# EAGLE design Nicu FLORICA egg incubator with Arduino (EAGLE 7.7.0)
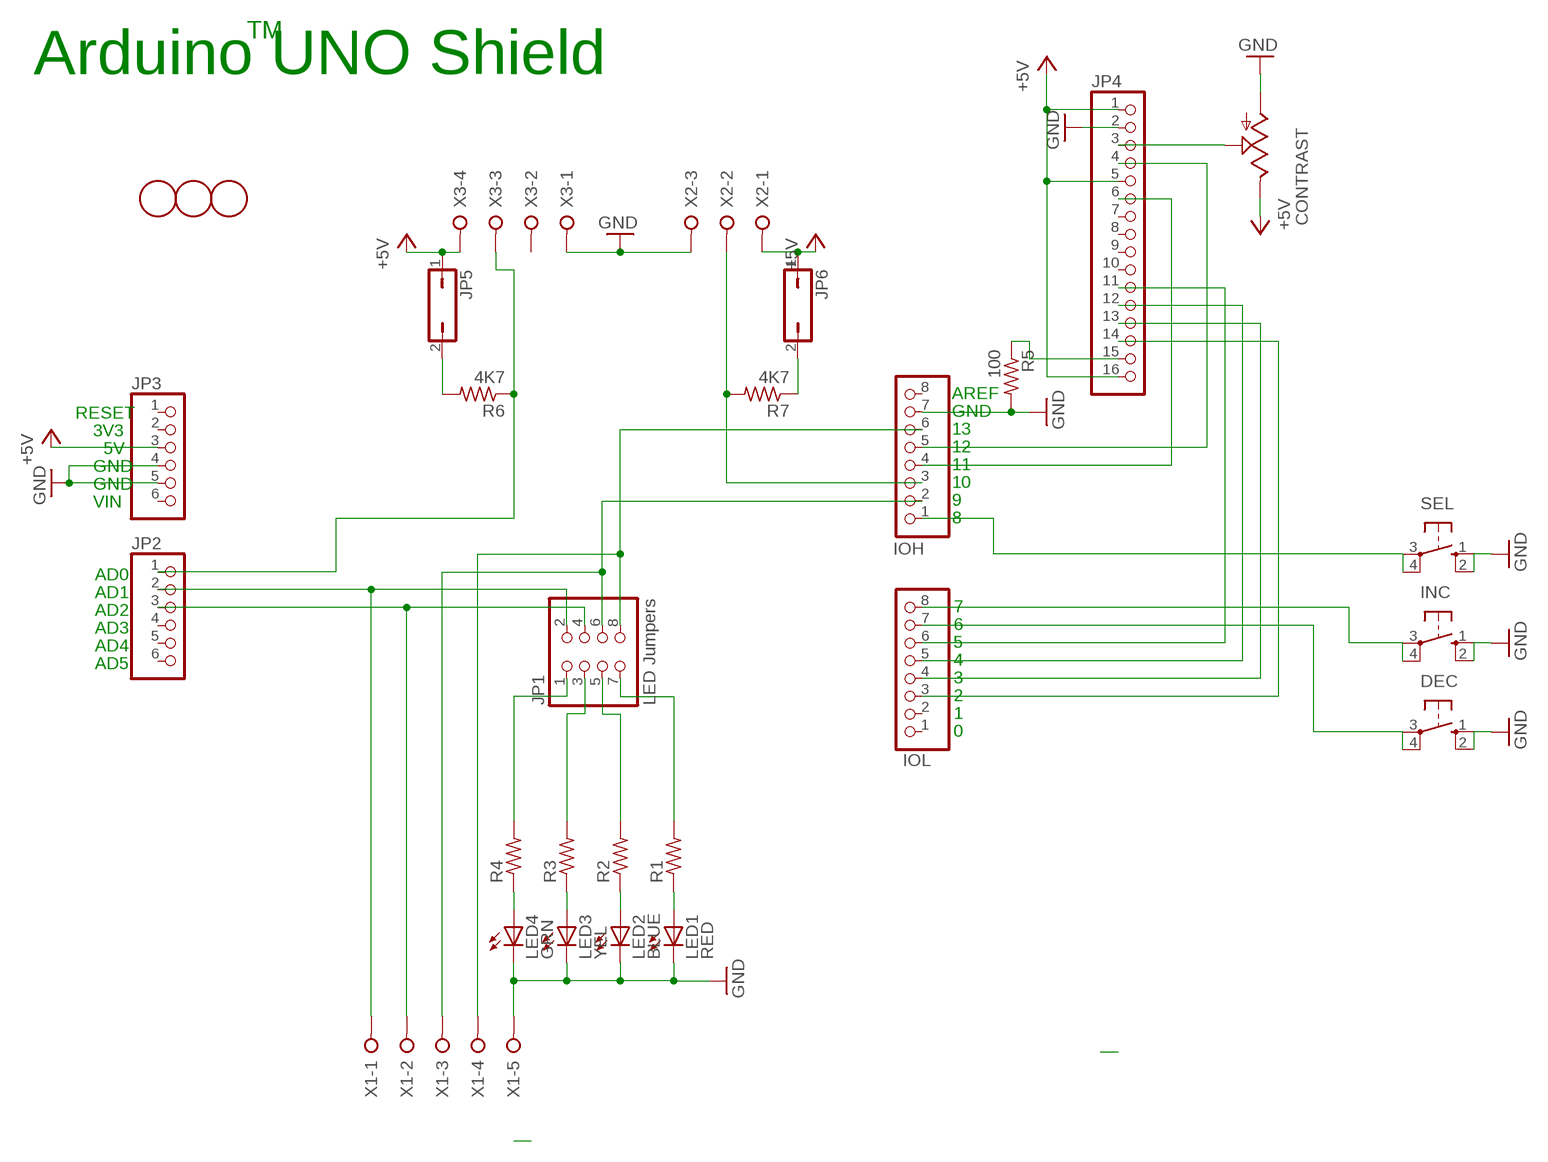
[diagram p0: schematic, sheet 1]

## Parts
CONTRAST  TRIM  [6MM]
DEC  10-XX  [B3F-10XX]
INC  10-XX  [B3F-10XX]
IOH  PINHD-1X8  [1X08]
IOL  PINHD-1X8  [1X08]
JP1  LED Jumpers  PINHD-2X4  [2X04]
JP2  PINHD-1X6  [1X06]
JP3  PINHD-1X6  [1X06]
JP4  PINHD-1X16  [1X16]
JP5  JP1Q  [JP1]
JP6  JP1Q  [JP1]
LED1  RED  LEDCHIPLED_0805  [CHIPLED_0805]
LED2  BLUE  LEDCHIPLED_0805  [CHIPLED_0805]
LED3  YEL  LEDCHIPLED_0805  [CHIPLED_0805]
LED4  GRN  LEDCHIPLED_0805  [CHIPLED_0805]
R1  R-US_R0805  [R0805]
R2  R-US_R0805  [R0805]
R3  R-US_R0805  [R0805]
R4  R-US_R0805  [R0805]
R5  100  R-US_R0805  [R0805]
R6  4K7  R-US_R0805  [R0805]
R7  4K7  R-US_R0805  [R0805]
SEL  10-XX  [B3F-10XX]
U$3  FIDUCIALMOUNT  [FIDUCIA-MOUNT]
U$4  FIDUCIALMOUNT  [FIDUCIA-MOUNT]
U$6  FIDUCIALMOUNT  [FIDUCIA-MOUNT]
X1  W237-05P  [W237-5P]
X2  W237-3E  [W237-3E]
X3  W237-04P  [W237-4P]

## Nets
+5V: CONTRAST.E JP3.3 JP4.1 JP4.5 JP4.16 JP5.1 JP6.1 X2.1 X3.4
GND: CONTRAST.A DEC.1(S) DEC.2(S1) INC.1(S) INC.2(S1) IOH.7 JP3.4 JP3.5 JP4.2 LED1.C LED2.C LED3.C LED4.C R5.2 SEL.1(S) SEL.2(S1) X1.5 X2.3 X3.1
N$1: IOH.6 JP1.8 X1.4
N$2: IOH.2 JP1.6 X1.3
N$3: JP1.4 JP2.3 X1.2
N$4: JP1.2 JP2.2 X1.1
N$5: LED1.A R1.1
N$6: LED2.A R2.1
N$8: LED3.A R3.1
N$9: LED4.A R4.1
N$10: CONTRAST.S JP4.3
N$11: JP4.15 R5.1
N$12: IOH.4 JP4.6
N$13: IOH.5 JP4.4
N$14: JP1.3 R3.2
N$15: JP1.5 R2.2
N$16: JP1.7 R1.2
N$17: JP1.1 R4.2
N$18: IOL.6 JP4.11
N$19: IOL.5 JP4.12
N$20: IOL.4 JP4.13
N$21: IOL.3 JP4.14
N$22: IOH.1 SEL.3(P) SEL.4(P1)
N$23: INC.3(P) INC.4(P1) IOL.8
N$24: DEC.3(P) DEC.4(P1) IOL.7
N$25: IOH.3 R7.2 X2.2
N$26: JP2.1 R6.1 X3.3
N$28: JP5.2 R6.2
N$29: JP6.2 R7.1
Unconnected: IOH.8 IOL.1 IOL.2 JP2.4 JP2.5 JP2.6 JP3.1 JP3.2 JP3.6 JP4.7 JP4.8 JP4.9 JP4.10 X3.2

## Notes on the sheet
- TM
- Arduino UNO Shield
- AREF
- RESET | GND
- 3V3 | 13
- 5V | 12
- GND | 11
- GND | 10
- VIN | 9
- 8
- AD0
- AD1
- AD2 | 7
- AD3 | 6
- AD4 | 5
- AD5 | 4
- 3
- 2
- 1
- 0

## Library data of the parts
CONTRAST = 1 New Library:TRIM
DEC INC SEL = 1 New Library:10-XX: OMRON SWITCH; MPN: B3F-1000; OC_FARNELL: 176432; OC_NEWARK: 36M3542
IOH IOL = 1 New Library:PINHD-1X8: PIN HEADER
JP1 = adafruit:PINHD-2X4: PIN HEADER
JP2 JP3 = pinhead:PINHD-1X6: PIN HEADER
JP4 = 1 New Library:PINHD-1X16: PIN HEADER
JP5 JP6 = jumper:JP1Q: JUMPER
LED1-LED4 = 1 New Library:LED: LED
R1-R7 = 1 New Library:R-US_: RESISTOR, American symbol
U$3 U$4 U$6 = SmartPrj:FIDUCIALMOUNT
X1 = con-wago-508:W237-05P: WAGO SREW CLAMP; OC_FARNELL: unknown; OC_NEWARK: unknown
X2 = con-wago-508:W237-3E: WAGO SREW CLAMP; OC_FARNELL: unknown; OC_NEWARK: unknown
X3 = con-wago-508:W237-04P: WAGO SREW CLAMP; OC_FARNELL: unknown; OC_NEWARK: unknown

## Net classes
0 default: width 0.152 mm, drill 0.305 mm, clearance 0.152 mm

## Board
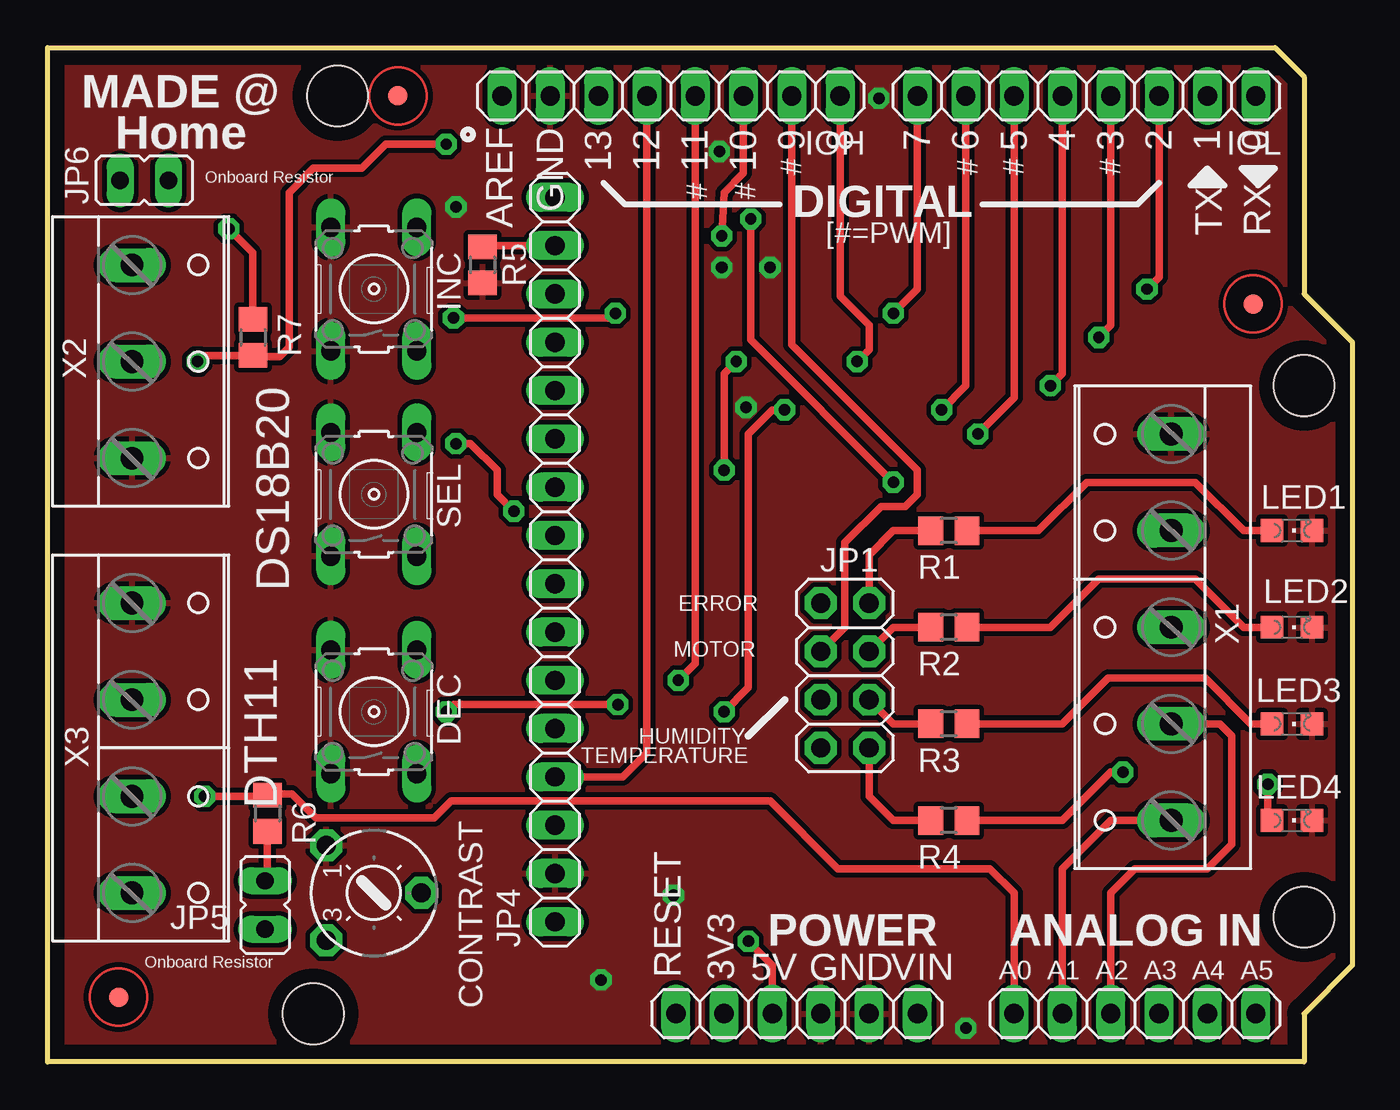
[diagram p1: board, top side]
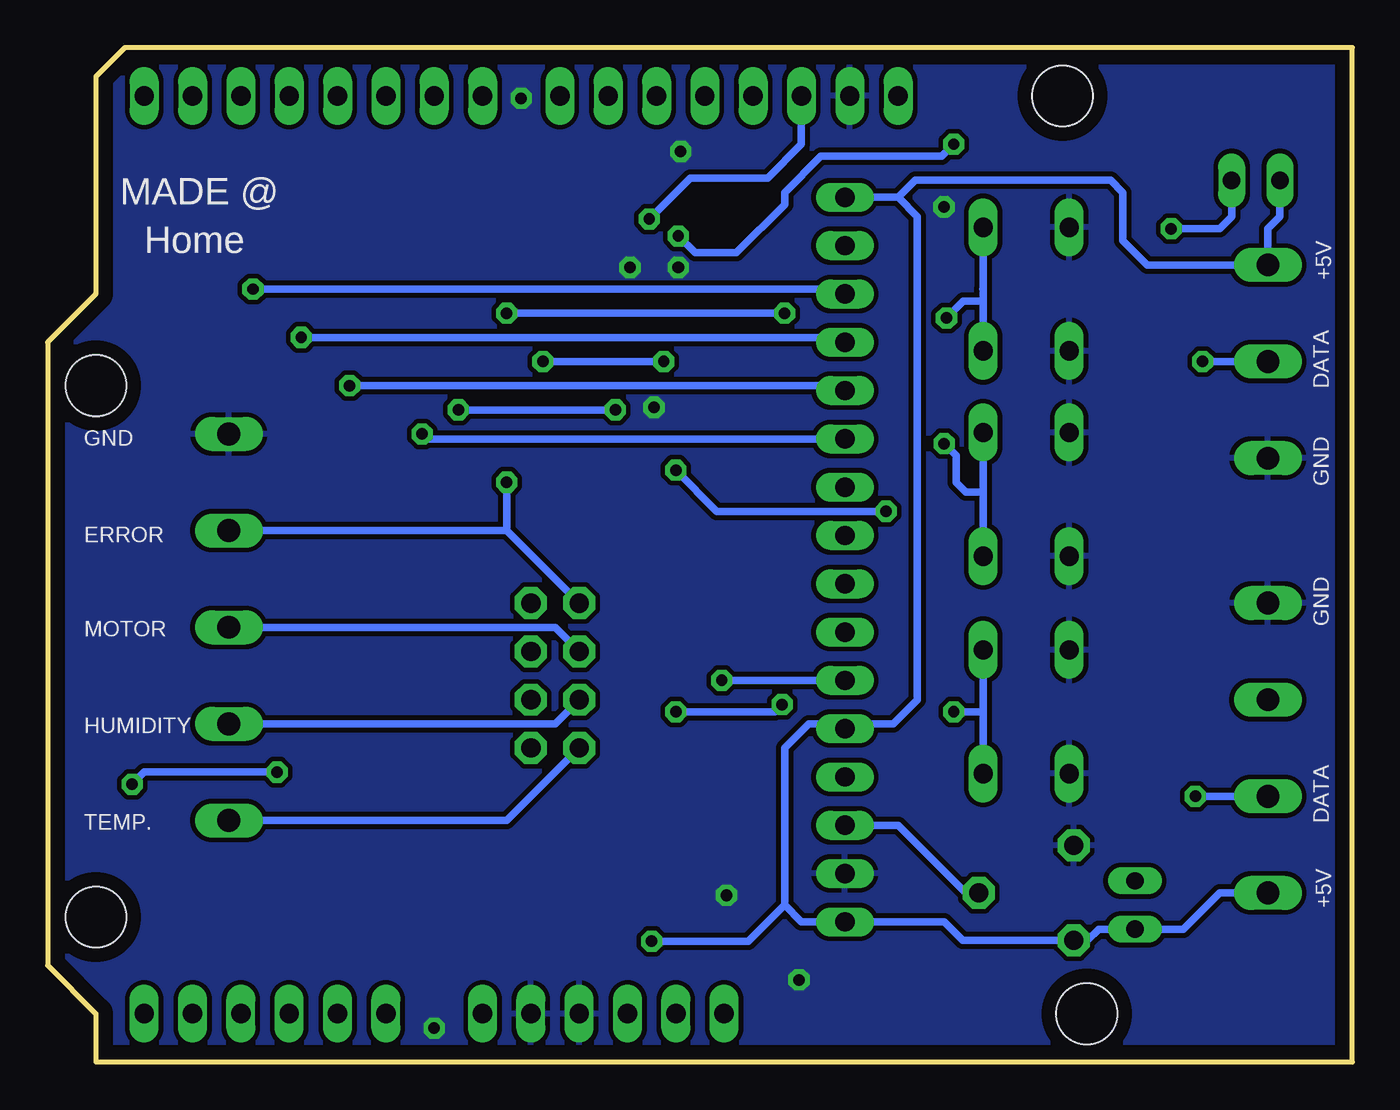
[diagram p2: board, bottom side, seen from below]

Size 68.58 x 53.34 mm. Coordinates in mm from the lower left corner, seen from the top.
Outline: 0,53.34 64.52,53.34 66.04,51.82 66.04,40.39 68.58,37.85 68.58,5.08 66.04,2.54 66.04,0 0,0 0,53.34
Copper layers (1*16): Top 0.035mm / dielectric 1.5mm / Bottom 0.035mm
Design rules "default *": minimum track width 8mil, minimum drill 12mil, track to track 6mil, track to pad 6mil, pad to pad 6mil, via to via 6mil, smd to smd 6mil, copper to edge 30mil, drill to drill 12mil, minimum pad ring 10mil, minimum via ring 10mil, stop-mask expansion 1mil, vias tented up to drill 0mil, thermal gap 10mil
Holes 3.2 mm at 66.04,35.56 66.04,7.62 15.24,50.8 13.97,2.54

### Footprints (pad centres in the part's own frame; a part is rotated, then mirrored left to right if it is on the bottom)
6MM = drill 1 pad 1.676 octagon: A -2.5,-2.5; E 2.5,-2.5; S 0,2.5
B3F-10XX = drill 1.016 long: 1 -3.251,2.261; 2 3.251,2.261; 3 -3.251,-2.261; 4 3.251,-2.261
1X08 = drill 1.016 long: 1 -8.89,0; 2 -6.35,0; 3 -3.81,0; 4 -1.27,0; 5 1.27,0; 6 3.81,0; 7 6.35,0; 8 8.89,0
2X04 = drill 1.016 pad 1.676 octagon: 1 -3.81,-1.27; 2 -3.81,1.27; 3 -1.27,-1.27; 4 -1.27,1.27; 5 1.27,-1.27; 6 1.27,1.27; 7 3.81,-1.27; 8 3.81,1.27
1X06 = drill 1.016 long: 1 -6.35,0; 2 -3.81,0; 3 -1.27,0; 4 1.27,0; 5 3.81,0; 6 6.35,0
1X16 = drill 1.016 long: 1 -19.05,0; 2 -16.51,0; 3 -13.97,0; 4 -11.43,0; 5 -8.89,0; 6 -6.35,0; 7 -3.81,0; 8 -1.27,0; 9 1.27,0; 10 3.81,0; 11 6.35,0; 12 8.89,0; 13 11.43,0; 14 13.97,0; 15 16.51,0; 16 19.05,0
JP1 = drill 0.914 long: 1 0,-1.27; 2 0,1.27
CHIPLED_0805 = smd 1.2 x 1.2: A 0,-1.05; C 0,1.05
R0805 = smd 1.3 x 1.5: 1 -0.95,0; 2 0.95,0
FIDUCIA-MOUNT = smd 1.016 x 1.016: P$1 0,0
W237-5P = drill 1.194 long: 1 -10.16,-0.635; 2 -5.08,-0.635; 3 0,-0.635; 4 5.08,-0.635; 5 10.16,-0.635
W237-3E = drill 1.194 long: 1 -5.08,-0.635; 2 0,-0.635; 3 5.08,-0.635
W237-4P = drill 1.194 long: 1 -7.62,-0.635; 2 -2.54,-0.635; 3 2.54,-0.635; 4 7.62,-0.635

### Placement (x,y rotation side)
CONTRAST  17.14,8.89 270 top
DEC  17.14,18.41 90 top
INC  17.14,40.64 90 top
IOH  32.77,50.8 180 top
IOL  54.61,50.8 180 top
JP1  41.91,20.32 90 top
JP2  57.15,2.54 0 top
JP3  39.37,2.54 0 top
JP4  26.67,26.42 90 top
JP5  11.43,8.26 0 top
JP6  5.08,46.35 270 top
LED1  65.41,27.94 270 top
LED2  65.41,22.86 270 top
LED3  65.41,17.78 270 top
LED4  65.41,12.7 270 top
R1  47.37,27.94 180 top
R2  47.37,22.86 180 top
R3  47.37,17.78 180 top
R4  47.37,12.7 180 top
R5  22.86,41.91 270 top
R6  11.56,13.08 270 top
R7  10.79,38.1 270 top
SEL  17.14,29.84 90 top
U$3  18.41,50.8 0 top
U$4  63.37,39.85 0 top
U$6  3.73,3.41 0 top
X1  58.42,22.86 90 top
X2  5.08,36.83 270 top
X3  5.08,16.51 270 top

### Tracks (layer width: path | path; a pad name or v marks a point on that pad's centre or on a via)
+5V  (via drill 0.6)
  Top 0.406: JP3.3 38.1,5.08 v36.83,6.35
  Bottom 0.406: JP4.16 23.88,45.47 | 23.88,45.47 22.86,44.45 22.86,19.05 24.13,17.78 26.42,17.78 JP4.5 26.92,17.78 28.57,17.78 29.84,16.51 29.84,8.26 | 29.84,8.26 28.96,7.37 JP4.1 21.46,7.37 20.49,6.39 CONTRAST.E 13.93,6.39 13.34,6.99 JP5.1 8.89,6.99 6.99,8.89 X3.4 | v36.83,6.35 31.75,6.35 29.84,8.26 | JP6.1 3.81,44.45 4.45,43.81 X2.1 10.79,41.91 12.06,43.18 12.06,45.72 12.7,46.35 22.99,46.35 23.88,45.47
GND  (via drill 0.61)
  other vias: 43.69,50.67 48.26,1.78 35.43,41.78 32.89,8.76 29.08,4.32 37.97,41.78 36.7,34.42 21.46,44.96 35.31,47.88
  pour Top (isolate 0.254): 0,53.34 68.58,53.34 68.58,0 0,0
  pour Bottom (isolate 0.254): 0,53.34 68.58,53.34 68.58,0 0,0
N$1  (via drill 0.6)
  Top 0.406: v36.96,44.32 36.96,37.97 v44.45,30.48
  Bottom 0.406: JP1.8 44.45,27.94 | 44.45,27.94 X1.4 | v44.45,30.48 44.45,27.94 | IOH.6 28.96,48.26 30.73,46.48 34.8,46.48 v36.96,44.32
N$2
  Top 0.406: IOH.2 39.12,37.72 45.72,31.11 45.72,29.84 45.09,29.21 43.81,29.21 41.91,27.3 41.91,22.86 JP1.6
  Bottom 0.406: X1.3 41.91,22.86 JP1.6
N$3
  Top 0.406: JP2.3 55.88,8.89 57.15,10.16 60.96,10.16 62.23,11.43 62.23,17.14 61.59,17.78 X1.2
  Bottom 0.406: JP1.4 41.91,17.78 X1.2
N$4
  Top 0.406: JP2.2 53.34,10.16 55.88,12.7 X1.1
  Bottom 0.406: JP1.2 44.45,12.7 X1.1
N$5
  Top 0.406: R1.1 52.07,27.94 54.61,30.48 60.33,30.48 62.87,27.94 LED1.A
N$6
  Top 0.406: R2.1 52.7,22.86 55.24,25.4 60.33,25.4 62.87,22.86 LED2.A
N$8
  Top 0.406: R3.1 53.34,17.78 55.75,20.19 60.83,20.19 63.25,17.78 LED3.A
N$9  (via drill 0.6)
  Top 0.406: R4.1 53.34,12.7 55.88,15.24 v56.52,15.24 | v64.14,14.61 64.14,12.92 LED4.A
  Bottom 0.406: v56.52,15.24 63.5,15.24 v64.14,14.61
N$10
  Bottom 0.406: JP4.3 23.88,12.45 20.32,8.89 CONTRAST.S
N$11
  Top 0.406: JP4.15 22.93,42.93 R5.1
N$12  (via drill 0.6)
  Top 0.406: IOH.4 34.04,20.95 v33.15,20.07
  Bottom 0.406: v33.15,20.07 JP4.6
N$13
  Top 0.406: IOH.5 31.5,16.26 30.23,14.99 JP4.4
N$14
  Top 0.406: JP1.3 44.45,17.78 R3.2
N$15
  Top 0.406: JP1.5 44.45,22.86 R2.2
N$16
  Top 0.406: JP1.7 43.18,26.67 44.45,27.94 R1.2
N$17
  Top 0.406: JP1.1 43.18,13.97 44.45,12.7 R4.2
N$18  (via drill 0.6)
  Top 0.406: IOL.6 50.8,34.92 v48.9,33.02
  Bottom 0.406: 26.92,33.02 JP4.11 48.64,32.77 v48.9,33.02
N$19  (via drill 0.6)
  Top 0.406: IOL.5 53.34,36.2 v52.7,35.56
  Bottom 0.406: v52.7,35.56 26.92,35.56 JP4.12
N$20  (via drill 0.6)
  Top 0.406: IOL.4 55.88,38.73 v55.24,38.1
  Bottom 0.406: v55.24,38.1 26.92,38.1 JP4.13
N$21  (via drill 0.6)
  Top 0.406: IOL.3 58.42,41.27 v57.78,40.64
  Bottom 0.406: v57.78,40.64 26.92,40.64 JP4.14
N$22  (via drill 0.6)
  Top 0.406: IOH.1 41.66,40.26 43.18,38.73 43.18,37.47 v42.55,36.83 | v36.2,36.83 35.56,36.2 v35.56,31.11 | v24.51,28.96 23.62,29.84 23.62,31.11 22.23,32.51 v21.46,32.51
  Bottom 0.406: SEL.3 19.41,29.97 | 19.41,29.97 SEL.4 | v42.55,36.83 v36.2,36.83 | v35.56,31.11 33.4,28.96 v24.51,28.96 | v21.46,32.51 20.83,31.88 20.83,30.48 20.32,29.97 19.41,29.97
N$23  (via drill 0.6)
  Top 0.406: IOL.8 45.72,40.64 v44.45,39.37 | v29.84,39.37 29.59,39.12 v21.34,39.12
  Bottom 0.406: INC.3 19.41,40.01 | 19.41,40.01 19.41,40.64 | 19.41,40.64 INC.4 | v44.45,39.37 v29.84,39.37 | 19.43,40.64 19.41,40.64 | v21.34,39.12 20.45,40.01 19.41,40.01
N$24  (via drill 0.6)
  Top 0.406: IOL.7 48.26,35.56 v46.99,34.29 | v38.73,34.29 38.1,34.29 36.83,33.02 36.83,19.68 v35.56,18.41 | v29.97,18.8 21.34,18.8 v20.95,18.41
  Bottom 0.406: DEC.3 19.41,18.41 | 19.41,18.41 DEC.4 | v46.99,34.29 v38.73,34.29 | v35.56,18.41 30.35,18.41 v29.97,18.8 | v20.95,18.41 19.41,18.41
N$25  (via drill 0.6)
  Top 0.406: v7.87,36.83 8.19,37.15 R7.2 10.86,37.08 12.19,37.08 12.7,37.59 12.7,45.72 13.97,46.99 16.51,46.99 17.78,48.26 v20.95,48.26 | IOH.3 36.58,46.74 35.56,45.72 v35.43,43.43
  Bottom 0.406: X2.2 v7.87,36.83 | v35.43,43.43 34.54,42.55 32.38,42.55 29.84,45.09 29.84,45.72 27.94,47.62 21.59,47.62 v20.95,48.26
N$26  (via drill 0.6)
  Top 0.406: v8.26,13.97 11.5,13.97 R6.1 11.62,14.1 12.83,14.1 14.1,12.83 20.32,12.83 21.21,13.72 37.97,13.72 41.53,10.16 49.53,10.16 50.8,8.89 JP2.1
  Bottom 0.406: v8.26,13.97 X3.3
N$27
  pour Top: 0.64,52.58 11.81,52.58 11.81,47.62 0.64,47.62
N$28
  Top 0.406: JP5.2 11.56,9.65 R6.2
N$29  (via drill 0.6)
  Top 0.406: R7.1 10.79,42.55 v9.53,43.81
  Bottom 0.406: v9.53,43.81 6.99,43.81 6.35,44.45 JP6.2

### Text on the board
tPlace: MADE @ | 13 | 12 | 11 | 10 | 9 | 8 | 7 | 6 | 5 | 4 | 3 | 2 | 1 | 0 | Home | Onboard Resistor | DS18B20 | ERROR | MOTOR | HUMIDITY | TEMPERATURE | DTH11 | Onboard Resistor
bPlace: +5V | DATA | GND | GND | ERROR | GND | MOTOR | HUMIDITY | DATA | TEMP. | +5V
tNames: AREF | GND | # | # | # | # | # | # | DIGITAL | [#=PWM] | TX | RX | POWER | ANALOG IN | RESET | 3V3 | 5V | GND | VIN | A0 | A1 | A2 | A3 | A4 | A5
bNames: MADE @ | Home
tDocu: Nicu FLORICA | Incubator
214bmp: D:/SmartProjects/Snc/a4_bn_logo2.bmp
